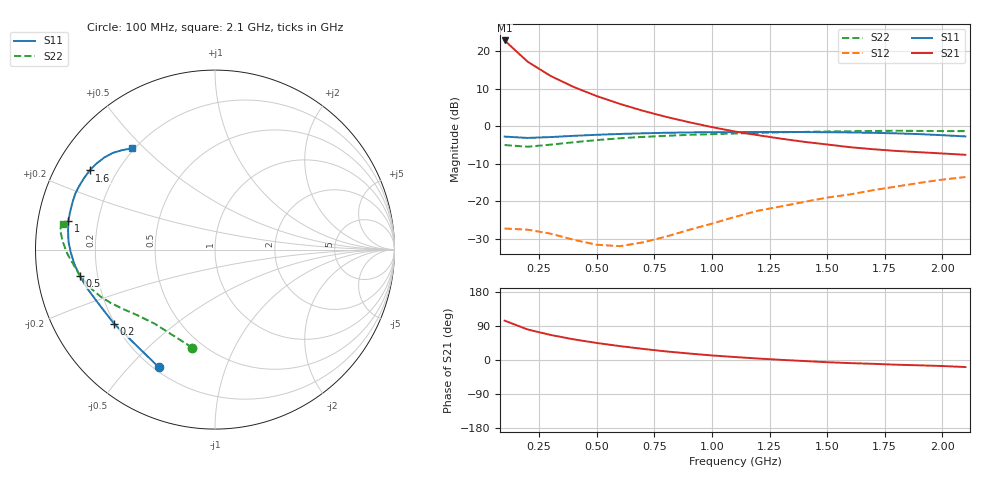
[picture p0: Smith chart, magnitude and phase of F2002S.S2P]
! Date: Fri Aug 11 13:12:59 1995
# MHZ  S  MA  R  50.0000
!  POLYFET RF DEVICES
!  F2002S
!  S PARAMETERS
!  VDS=28V, IDQ=400mA
! FREQ  S11MAG  S11ANG  S21MAG  S21ANG  S12MAG  S12ANG  S22MAG  S22ANG
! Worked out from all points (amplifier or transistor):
!   21 points, 100 MHz to 2.1 GHz, reference 50 ohm
!   highest |S21| = 22.8 dB at 100 MHz (marker M1)
!   |S21| within 3 dB of that: start of sweep to 153 MHz
!   unconditionally stable (mu >= 1): 410 MHz to 1.087 GHz
!   at 400 MHz: K = 0.97, MSG = 20.4 dB, |S12| = -30.3 dB
!   at 1.1 GHz: K = 0.98, MSG = 11.4 dB, |S12| = -24.2 dB
!   at 2.1 GHz: K = 0.61, MSG = 3.0 dB, |S12| = -13.6 dB
!   S11 on the Smith chart (normalised r, x): 100 MHz: 0.22, -0.61; 200 MHz: 0.20, -0.32; 500 MHz: 0.13, -0.09; 1 GHz: 0.09, +0.10; 1.6 GHz: 0.10, +0.29; 2.1 GHz: 0.19, +0.46
100  0.7267 -115.4  13.87 103.9  0.04333 20.6  0.5609 -103.0
200  0.6976 -143.6  7.225 80.6  0.04184 5.2  0.5324 -129.1
300  0.7163 -155.4  4.663 66.0  0.03702 -0.0  0.5678 -140.1
400  0.7442 -163.1  3.328 54.5  0.03063 3.5  0.611 -147.3
500  0.7683 -169.1  2.518 44.9  0.02635 12.3  0.6531 -153.0
600  0.7881 -174.2  1.983 36.7  0.02522 29.3  0.6899 -157.8
700  0.8037 -178.9  1.606 29.4  0.02834 43.2  0.7203 -162.1
800  0.8175 176.8  1.333 22.7  0.03375 55.4  0.7436 -166.0
900  0.8255 172.6  1.131 17.1  0.04156 60.7  0.7671 -169.4
1000  0.8326 168.9  0.9719 12.0  0.05034 64.6  0.7839 -172.3
1100  0.8344 165.2  0.8493 7.9  0.06195 64.9  0.7989 -175.0
1200  0.8365 161.6  0.7582 3.9  0.07486 65.1  0.8136 -177.0
1300  0.8384 158.1  0.6822 0.4  0.0854 63.3  0.8288 -179.3
1400  0.8351 154.6  0.6188 -2.7  0.09795 60.8  0.839 178.7
1500  0.831 151.1  0.5708 -5.8  0.1119 57.5  0.85 177.0
1600  0.826 147.7  0.5246 -8.2  0.1235 56.8  0.8571 175.3
1700  0.8159 144.0  0.4933 -10.1  0.1404 53.3  0.8634 174.0
1800  0.8028 140.4  0.468 -12.4  0.1571 50.4  0.87 172.8
1900  0.7844 136.6  0.4503 -14.1  0.1757 45.5  0.8657 171.2
2000  0.7585 133.1  0.4332 -15.9  0.1942 40.9  0.86 170.5
2100  0.7307 129.5  0.416 -18.6  0.2101 35.9  0.8588 170.3
